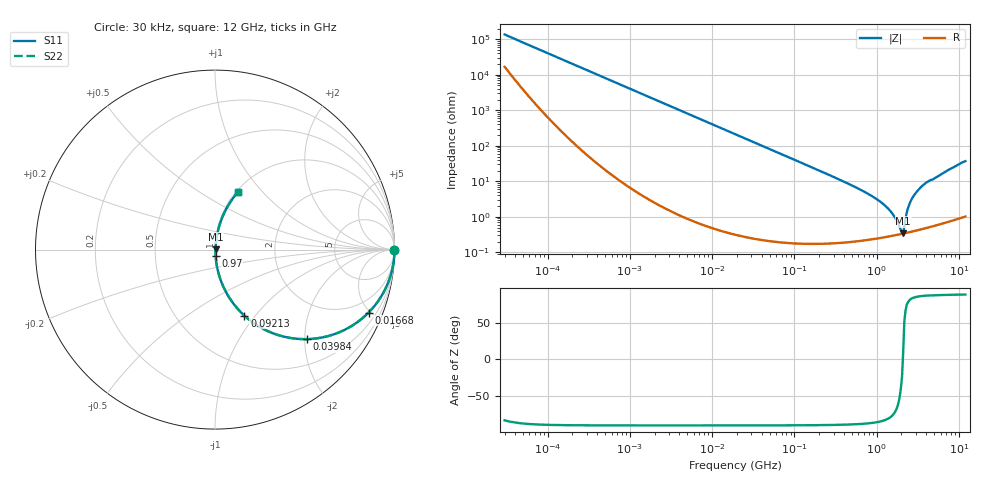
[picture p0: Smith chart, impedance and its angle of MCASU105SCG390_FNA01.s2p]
! MCASU105SCG390_FNA01  S-PARAMETER MODEL  ( General Type )
! Model Generated by TAIYO YUDEN Corporation (http://www.ty-top.com)
! Version 1.0
! TAIYO YUDEN Control No. 130207
! Copyright(c) 2013 TAIYO YUDEN CO.,LTD. All Rights Reserved.
! Product Description (link to TY-COMPAS)
! https://ds.yuden.co.jp/TYCOMPAS/or/detail?pn=MCASU105SCG390JFNA01&u=M
! Products Name : Multilayer Ceramic Capacitors
! Characteristics :
!  Capacitance : 39 pF , Rated Voltage : 50V , TCC : CG / C0G
!  Case Size : 1.0 x 0.5 / 0.039 x 0.02 [mm/inch] , Thickness : 0.5 / 0.02 [mm/inch]
!  (Conditions: Temperature = 25 degC , DC Bias Current/Voltage = 0A / 0V)
! External Node Assignments :
!  1  o---| |---o  2
! GND o---------o GND
! Frequency Range : 30000Hz  -  12GHz  [ 401 STEP ]
# MHz S RI R 50
! Freq[MHz].  S11 Real  S11 Imag  S21 Real  S21 Imag  S12 Real  S12 Imag  S22 Real  S22 Imag
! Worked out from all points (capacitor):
!   401 points, 30 kHz to 12 GHz, reference 50 ohm
!   read as one part in series: C = 39.2 pF near 32 kHz
!   lowest |Z| = 343 mohm at 2.103 GHz (marker M1)
!   series resonance near 2.084 GHz, so ESL is about 150 pH
!   S11 on the Smith chart (normalised r, x): 30 kHz: open; 16.68 MHz: 1.01, -4.87; 39.84 MHz: 1.00, -2.04; 92.13 MHz: 1.00, -0.88; 970 MHz: 1.00, -0.07; 12 GHz: 1.02, +0.74
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0.03  0.9999 -0.000727  9.07e-05 0.000727  9.07e-05 0.000727  0.9999 -0.000727
0.260295  0.9999 -0.0064  7.13e-05 0.0064  7.13e-05 0.0064  0.9999 -0.0064
2.258455  0.9969 -0.0554  0.00314 0.0554  0.00314 0.0554  0.9969 -0.0554
6.54608  0.9745 -0.157  0.0255 0.157  0.0255 0.157  0.9745 -0.157
16.67749  0.8555 -0.3509  0.1445 0.3509  0.1445 0.3509  0.8555 -0.3509
18.97367  0.8206 -0.3829  0.1794 0.3829  0.1794 0.3829  0.8206 -0.3829
39.83545  0.5098 -0.4988  0.4902 0.4988  0.4902 0.4988  0.5098 -0.4988
92.13054  0.1634 -0.3677  0.8366 0.3677  0.8366 0.3677  0.1634 -0.3677
164.6252  0.0582 -0.2307  0.9418 0.2307  0.9418 0.2307  0.0582 -0.2307
508.9517  0.00757 -0.0745  0.9924 0.0745  0.9924 0.0745  0.00757 -0.0745
970.0175  0.00349 -0.0329  0.9965 0.0329  0.9965 0.0329  0.00349 -0.0329
1428.372  0.00305 -0.0154  0.997 0.0154  0.997 0.0154  0.00305 -0.0154
1678.29  0.0031 -0.00891  0.9969 0.00891  0.9969 0.00891  0.0031 -0.00891
1971.936  0.00327 -0.00267  0.9967 0.00267  0.9967 0.00267  0.00327 -0.00267
2103.309  0.00337 0.0006  0.9966 -0.0006  0.9966 -0.0006  0.00337 0.0006
2172.242  0.00344 0.00435  0.9966 -0.00435  0.9966 -0.00435  0.00344 0.00435
2392.896  0.00387 0.0163  0.9961 -0.0163  0.9961 -0.0163  0.00387 0.0163
2552.314  0.00435 0.0249  0.9957 -0.0249  0.9957 -0.0249  0.00435 0.0249
2811.574  0.00539 0.0382  0.9946 -0.0382  0.9946 -0.0382  0.00539 0.0382
3303.507  0.00797 0.0604  0.992 -0.0604  0.992 -0.0604  0.00797 0.0604
4275.791  0.0149 0.0986  0.9851 -0.0986  0.9851 -0.0986  0.0149 0.0986
12000  0.1273 0.3199  0.8727 -0.3199  0.8727 -0.3199  0.1273 0.3199
